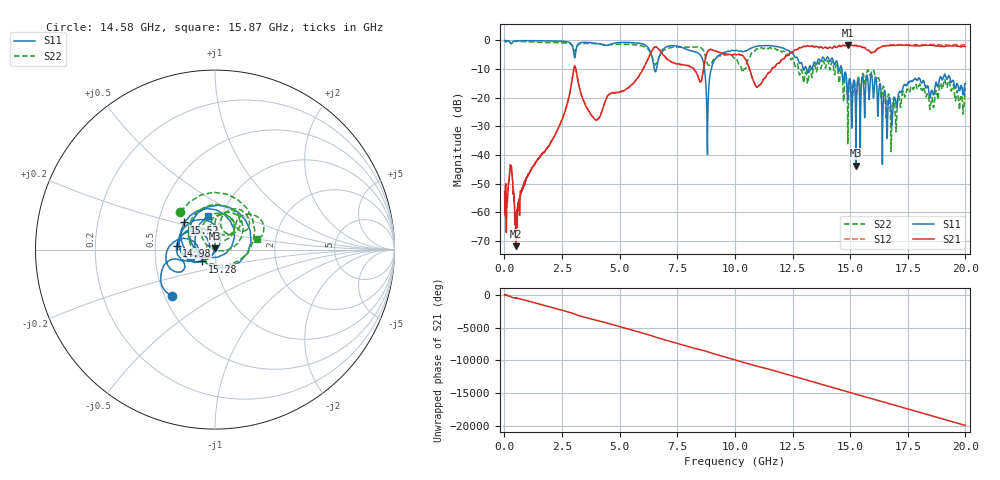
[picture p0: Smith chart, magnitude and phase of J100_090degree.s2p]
!Keysight Technologies,N5222A,MY51421036,A.10.65.16
!Date: Friday, March 31, 2023 14:45:13
!Correction: S11(Full 2 Port(1,2))
!S21(Full 2 Port(1,2))
!S12(Full 2 Port(1,2))
!S22(Full 2 Port(1,2))
!S2P File: Measurements: S11, S21, S12, S22:
# Hz S  dB  R 50
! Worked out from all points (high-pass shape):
!   2000 points, 10 MHz to 20 GHz, reference 50 ohm
!   highest |S21| = -1.60 dB at 14.91 GHz (marker M1); lowest = -71.9 dB at 490 MHz (marker M2)
!   |S21| within 3 dB of the highest: 8.774 GHz to 9.463 GHz (689.3 MHz wide, 7.56 % of centre); 12.38 GHz to end of sweep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
!   lowest |S11| = -43.7 dB at 15.25 GHz (marker M3), VSWR 1.01, Z = 50.1 + j0.649 ohm
!   |S11| at or under -10 dB: 8.681 GHz to 8.975 GHz (294.4 MHz wide, 3.33 % of centre); 13.11 GHz to 13.21 GHz (97.82 MHz wide, 0.744 % of centre); 14.64 GHz to end of sweep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
!   |S22| runs from -38.8 to -0.1 dB; largest |S21 - S12| = 0.064
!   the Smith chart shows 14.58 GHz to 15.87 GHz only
!   S11 on the Smith chart (normalised r, x): 14.58 GHz: 0.55, -0.32; 14.98 GHz: 0.65, +0.03; 15.28 GHz: 0.86, -0.11; 15.52 GHz: 0.68, +0.22; 15.87 GHz: 0.86, +0.34
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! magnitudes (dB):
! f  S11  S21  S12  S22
! 10 MHz  0.0  -52.8  -61.5  -0.1
! 270 MHz  -1.1  -44.0  -44.0  -0.2
! 490 MHz  -0.2  -71.9  -62.5  -0.3
! 3.03 GHz  -5.4  -9.2  -9.2  -3.7
! 3.35 GHz  -0.8  -19.4  -19.3  -1.1
! 4.04 GHz  -1.1  -27.6  -27.5  -1.2
! 6.68 GHz  -6.7  -2.9  -2.8  -6.2
! 8.43 GHz  -4.5  -13.3  -13.3  -2.3
! 8.82 GHz  -29.0  -3.8  -3.8  -8.2
! 9.12 GHz  -6.8  -3.6  -3.5  -6.4
! 10.01 GHz  -3.6  -4.9  -4.9  -6.2
! 10.99 GHz  -2.0  -16.2  -16.2  -3.0
! 13.34 GHz  -10.2  -1.9  -1.8  -13.0
! 14.58 GHz  -9.1  -2.1  -2.0  -10.9
! 14.91 GHz  -19.1  -1.6  -1.5  -32.0
! 14.98 GHz  -13.3  -1.8  -1.7  -13.9
! 15.25 GHz  -43.7  -1.8  -1.7  -19.8
! 15.28 GHz  -20.2  -1.9  -1.7  -19.3
! 15.52 GHz  -12.9  -2.5  -2.3  -12.6
! 15.87 GHz  -14.3  -4.1  -4.0  -12.3
! 16.67 GHz  -21.1  -1.8  -1.6  -18.7
! 20 GHz  -15.1  -2.1  -1.6  -16.7
